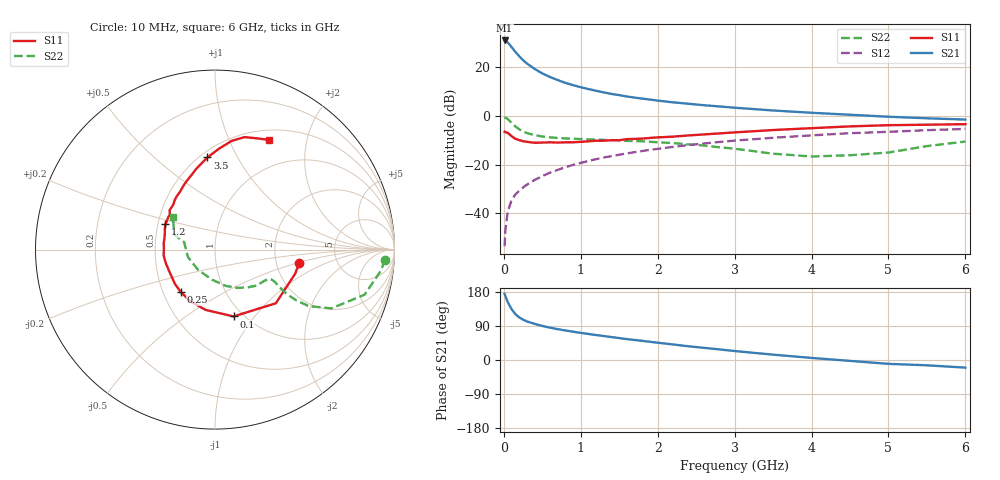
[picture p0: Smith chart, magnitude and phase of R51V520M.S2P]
! SIEMENS Small Signal Semiconductors
! BFR183
! Si NPN RF Bipolar Junction Transistor in SOT23
! VCE = 1.5 V  IC = 20 mA
! Common Emitter S-Parameters:  May  1996
# GHz  S  MA  R  50
!  f  S11  S21  S12  S22
! GHz  MAG  ANG  MAG  ANG  MAG  ANG  MAG  ANG
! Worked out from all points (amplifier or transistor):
!   36 points, 10 MHz to 6 GHz, reference 50 ohm
!   highest |S21| = 31.1 dB at 10 MHz (marker M1)
!   |S21| within 3 dB of that: start of sweep to 108.2 MHz
!   unconditionally stable (mu >= 1): 473.6 MHz to 2.457 GHz
!   at 250 MHz: K = 0.84, MSG = 26.2 dB, |S12| = -29.4 dB
!   at 1.4 GHz: K = 1.06, MAG = 11.3 dB, |S12| = -16.5 dB
!   at 6 GHz: K = 0.92, MSG = 1.9 dB, |S12| = -5.3 dB
!   S11 on the Smith chart (normalised r, x): 10 MHz: 2.70, -0.52; 100 MHz: 0.90, -0.79; 250 MHz: 0.62, -0.32; 1.2 GHz: 0.55, +0.17; 3.5 GHz: 0.54, +0.76; 6 GHz: 0.62, +1.41
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0.01  0.4755 -9.1  35.91 174.3  0.0021 87.8  0.9481 -3.4
0.02  0.466 -16.9  35.51 168.5  0.0045 79.7  0.9321 -7.2
0.05  0.4521 -41.4  32.91 153.3  0.0107 76.0  0.8703 -16.8
0.1  0.3865 -74.5  26.42 134.1  0.0185 70.1  0.7265 -26.8
0.15  0.3401 -98.7  20.91 121.0  0.0244 65.7  0.609 -31.1
0.2  0.3193 -115.4  17.02 112.6  0.0289 66.2  0.5341 -32.0
0.25  0.3036 -128.8  14.11 106.4  0.0338 66.5  0.4812 -31.8
0.3  0.2941 -139.1  12.05 101.8  0.0388 68.2  0.4465 -31.2
0.4  0.2824 -154.0  9.328 95.4  0.0483 69.4  0.4041 -29.6
0.5  0.2843 -164.6  7.541 89.9  0.058 70.2  0.3793 -28.4
0.6  0.2882 -173.7  6.35 85.4  0.0684 70.6  0.3645 -28.0
0.7  0.2844 179.2  5.492 81.4  0.0779 70.5  0.3543 -28.0
0.8  0.2878 173.2  4.821 77.9  0.0884 70.0  0.3463 -28.3
0.9  0.2885 167.6  4.319 74.7  0.0988 69.5  0.3405 -28.7
1.1  0.302 157.8  3.591 68.8  0.119 68.5  0.3315 -30.9
1.2  0.3107 153.0  3.309 65.8  0.1297 67.8  0.3262 -31.9
1.6  0.335 139.1  2.526 55.1  0.1704 63.7  0.3083 -38.1
2.2  0.3768 121.2  1.914 41.0  0.2322 57.2  0.2776 -49.8
3.5  0.5152 94.7  1.301 14.1  0.3568 39.9  0.1679 -96.0
4.5  0.6125 81.3  1.063 -2.3  0.4437 26.7  0.1561 -164.5
5.5  0.6631 69.2  0.899 -14.0  0.5118 14.7  0.2409 159.9
6  0.6801 64.0  0.846 -20.1  0.5429 7.0  0.2984 142.0
